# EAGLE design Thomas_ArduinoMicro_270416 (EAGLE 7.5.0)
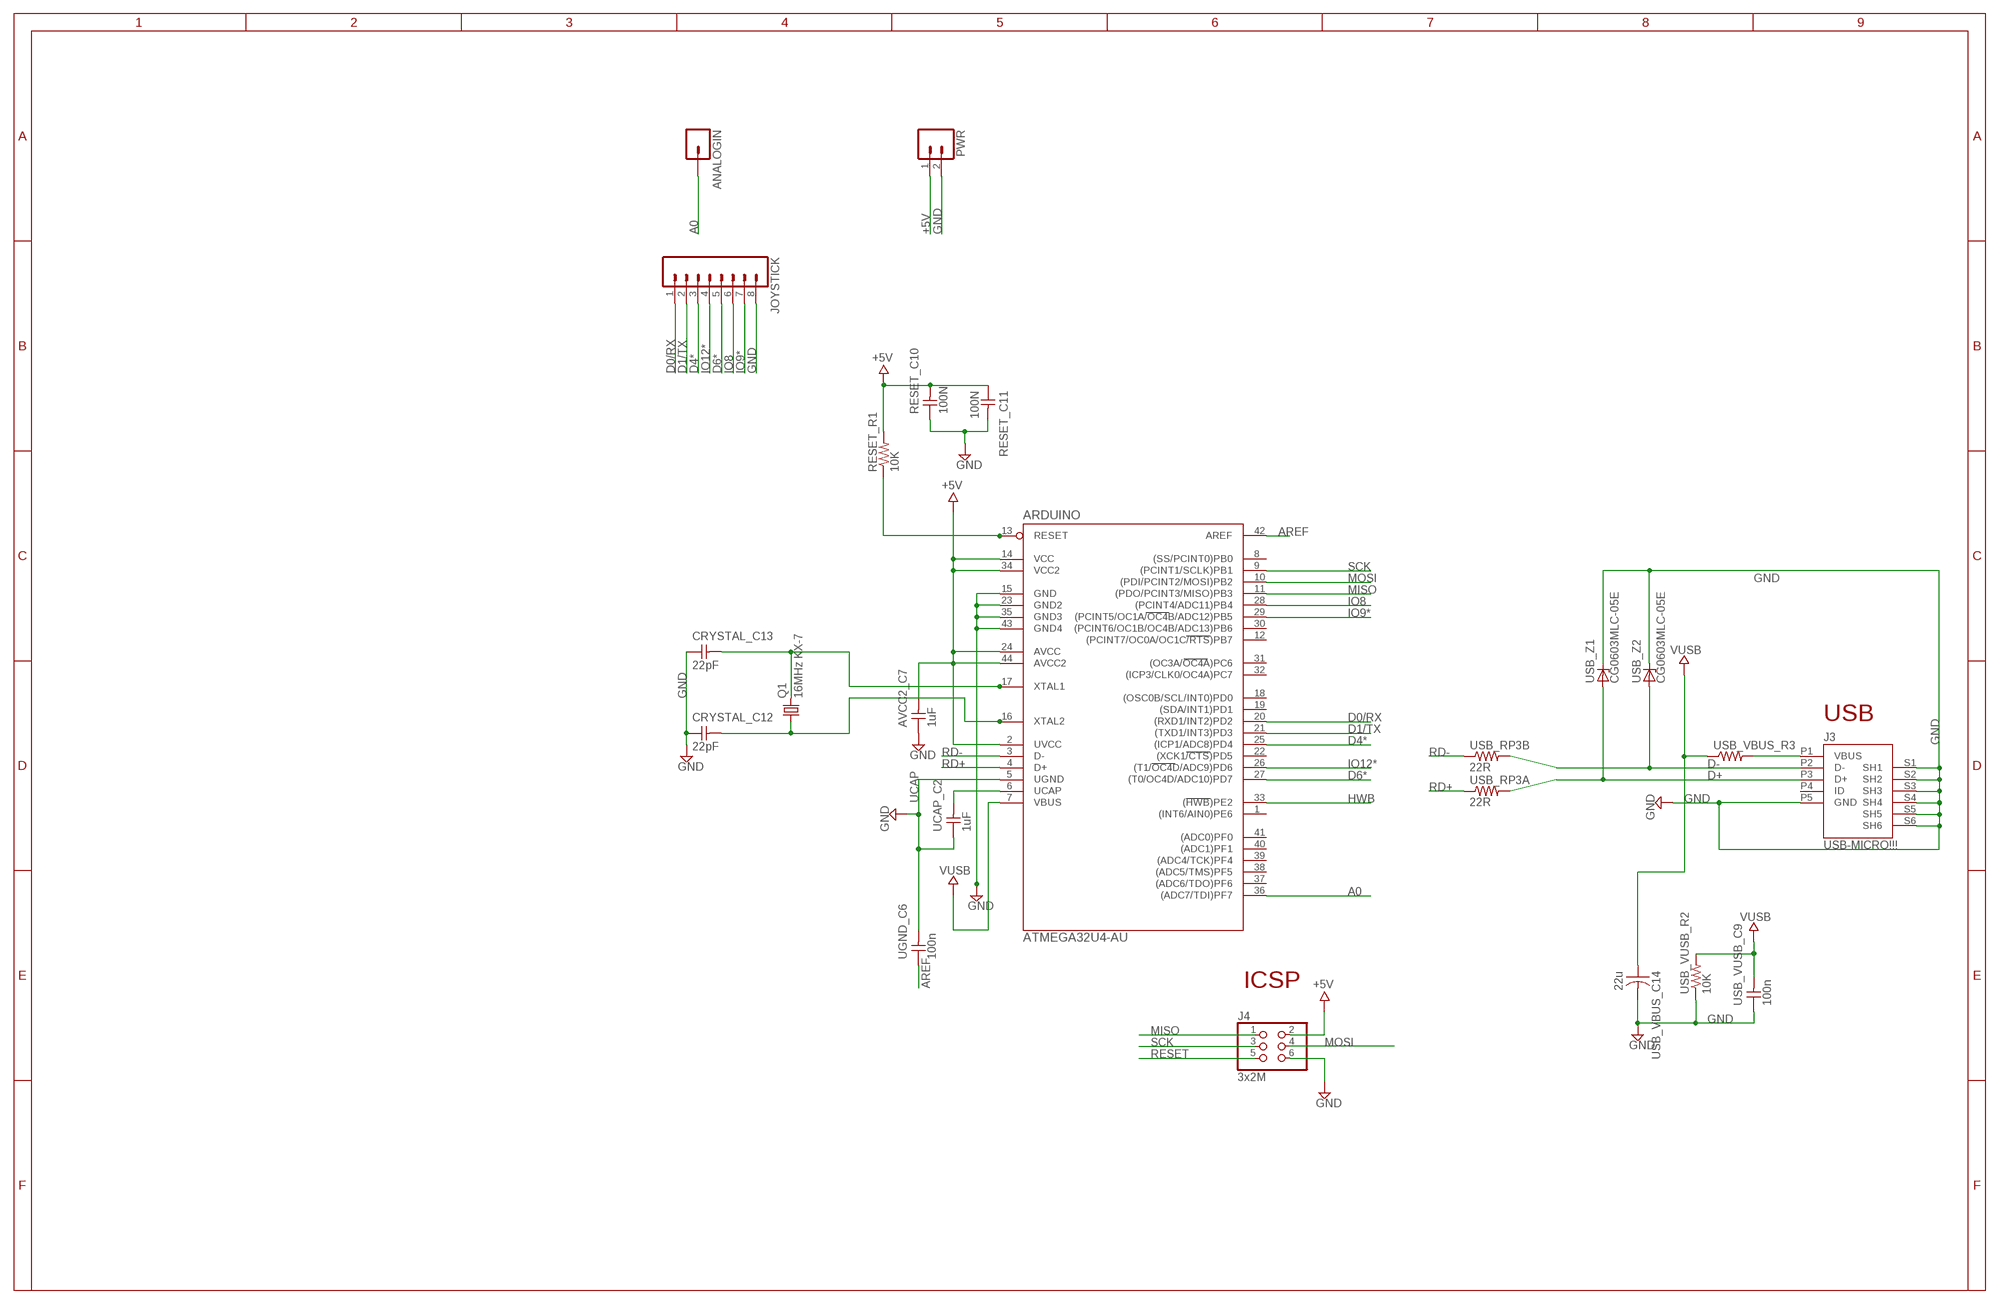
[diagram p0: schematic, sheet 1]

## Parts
ANALOGIN  M01PTH_LONGPAD  [1X01_LONGPAD]
ARDUINO  ATMEGA32U4-AU  [TQFP44]
AVCC2_C7  1uF  CAP-UNPOLARIZEDFAB  [C1206FAB]
CRYSTAL_C12  22pF  CAP-UNPOLARIZEDFAB  [C1206FAB]
CRYSTAL_C13  22pF  CAP-UNPOLARIZEDFAB  [C1206FAB]
J3  USB-MICRO!!!  MYCON2_USB-MINI-B  [CON2_USB_MICRO_B_AT]
J4  3x2M  PINHD-2X3  [2X03]
JOYSTICK  M08LONGPADS  [1X08_LONGPADS]
PWR  M02PTH3  [1X02_LONGPADS]
Q1  16MHz KX-7  CSM-7X-DU  [CSM-7X-DU]
RESET_C10  100N  CAP-UNPOLARIZEDFAB  [C1206FAB]
RESET_C11  100N  CAP-UNPOLARIZEDFAB  [C1206FAB]
RESET_R1  10K  RESISTOR1206  [1206]
UCAP_C2  1uF  CAP-UNPOLARIZEDFAB  [C1206FAB]
UGND_C6  100n  CAP-UNPOLARIZEDFAB  [C1206FAB]
USB_RP3A  22R  RESISTOR1206  [1206]
USB_RP3B  22R  RESISTOR1206  [1206]
USB_VBUS_C14  22u  CAP-US1206FAB  [C1206FAB]
USB_VBUS_R3  RESISTOR1206  [1206]
USB_VUSB_C9  100n  CAP-UNPOLARIZEDFAB  [C1206FAB]
USB_VUSB_R2  10K  RESISTOR1206  [1206]
USB_Z1  CG0603MLC-05E  ZENER_DIODESOD123  [SOD123]
USB_Z2  CG0603MLC-05E  ZENER_DIODESOD123  [SOD123]

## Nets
+5V: ARDUINO.2(UVCC) ARDUINO.14(VCC) ARDUINO.24(AVCC) ARDUINO.34(VCC2) ARDUINO.44(AVCC2) AVCC2_C7.2 J4.2 PWR.1
A0: ANALOGIN.1 ARDUINO.36((ADC7/TDI)PF7)
AREF: ARDUINO.42(AREF) UGND_C6.1
C11: RESET_C10.2 RESET_C11.1 RESET_R1.2 ; supply symbol labelled +5V
D0/RX: ARDUINO.20((RXD1/INT2)PD2) JOYSTICK.1
D1/TX: ARDUINO.21((TXD1/INT3)PD3) JOYSTICK.2
D4*: ARDUINO.25((ICP1/ADC8)PD4) JOYSTICK.3
D6*: ARDUINO.27((T0/OC4D/ADC10)PD7) JOYSTICK.5
D+: J3.P3(D+) USB_RP3A.2 USB_Z1.ANODE
D-: J3.P2(D-) USB_RP3B.2 USB_Z2.ANODE
GND: ARDUINO.15(GND) ARDUINO.23(GND2) ARDUINO.35(GND3) ARDUINO.43(GND4) AVCC2_C7.1 CRYSTAL_C12.1 CRYSTAL_C13.1 J3.P5(GND) J3.S1(SH1) J3.S2(SH2) J3.S3(SH3) J3.S4(SH4) J3.S5(SH5) J3.S6(SH6) J4.6 JOYSTICK.8 PWR.2 RESET_C10.1 RESET_C11.2 USB_VBUS_C14.2 USB_VUSB_C9.1 USB_VUSB_R2.1 USB_Z1.CATHODE USB_Z2.CATHODE
HWB: ARDUINO.33((HWB)PE2)
IO8: ARDUINO.28((PCINT4/ADC11)PB4) JOYSTICK.6
IO9*: ARDUINO.29((PCINT5/OC1A/OC4B/ADC12)PB5) JOYSTICK.7
IO12*: ARDUINO.26((T1/OC4D/ADC9)PD6) JOYSTICK.4
MISO: ARDUINO.11((PDO/PCINT3/MISO)PB3) J4.1
MOSI: ARDUINO.10((PDI/PCINT2/MOSI)PB2) J4.4
N$1: ARDUINO.13(RESET) RESET_R1.1
N$2: ARDUINO.6(UCAP) UCAP_C2.2
N$3: ARDUINO.16(XTAL2) CRYSTAL_C12.2 Q1.1
N$4: ARDUINO.17(XTAL1) CRYSTAL_C13.2 Q1.2
N$5: J3.P1(VBUS) USB_VBUS_R3.2
RD+: ARDUINO.4(D+) USB_RP3A.1
RD-: ARDUINO.3(D-) USB_RP3B.1
RESET: J4.5
SCK: ARDUINO.9((PCINT1/SCLK)PB1) J4.3
UCAP: ARDUINO.5(UGND) UCAP_C2.1 UGND_C6.2 ; supply symbol labelled GND
VUSB: ARDUINO.7(VBUS) USB_VBUS_C14.1 USB_VBUS_R3.1 USB_VUSB_C9.2 USB_VUSB_R2.2
Unconnected: ARDUINO.1((INT6/AIN0)PE6) ARDUINO.8((SS/PCINT0)PB0) ARDUINO.12((PCINT7/OC0A/OC1C/RTS)PB7) ARDUINO.18((OSC0B/SCL/INT0)PD0) ARDUINO.19((SDA/INT1)PD1) ARDUINO.22((XCK1/CTS)PD5) ARDUINO.30((PCINT6/OC1B/OC4B/ADC13)PB6) ARDUINO.31((OC3A/OC4A)PC6) ARDUINO.32((ICP3/CLK0/OC4A)PC7) ARDUINO.37((ADC6/TDO)PF6) ARDUINO.38((ADC5/TMS)PF5) ARDUINO.39((ADC4/TCK)PF4) ARDUINO.40((ADC1)PF1) ARDUINO.41((ADC0)PF0) J3.P4(ID)

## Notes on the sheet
- USB
- ICSP

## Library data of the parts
ANALOGIN = SparkFun-Connectors:M01: Header 1
ARDUINO = mega32U4:ATMEGA32U4-AU
AVCC2_C7 CRYSTAL_C12 CRYSTAL_C13 RESET_C10 RESET_C11 UCAP_C2 UGND_C6 USB_VUSB_C9 = fab:CAP-UNPOLARIZED
J3 = SmartPrj:MYCON2_USB-MINI-B
J4 = SmartPrj:PINHD-2X3: PIN HEADER
JOYSTICK = SparkFun-Connectors:M08: Header 8 Standard 8-pin 0.1" header. Use with straight break away headers (SKU : PRT-00116), right angle break away headers (PRT-00553), swiss pins (PRT-00743), machine pins (PRT-00117), and female headers (PRT-00115).
PWR = SparkFun-Connectors:M02: Standard 2-pin 0.1" header. Use with
Q1 = FAB_Hello:CSM-7X-DU: SMD CRYSTAL; OC_FARNELL: unknown; OC_NEWARK: unknown
RESET_R1 USB_RP3A USB_RP3B USB_VBUS_R3 USB_VUSB_R2 = SparkFun-Passives:RESISTOR: Resistor
USB_VBUS_C14 = fab:CAP-US
USB_Z1 USB_Z2 = fab:ZENER_DIODE: zener diode

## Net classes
0 default: width 0.254 mm, drill 0.61 mm, clearance 0.203 mm

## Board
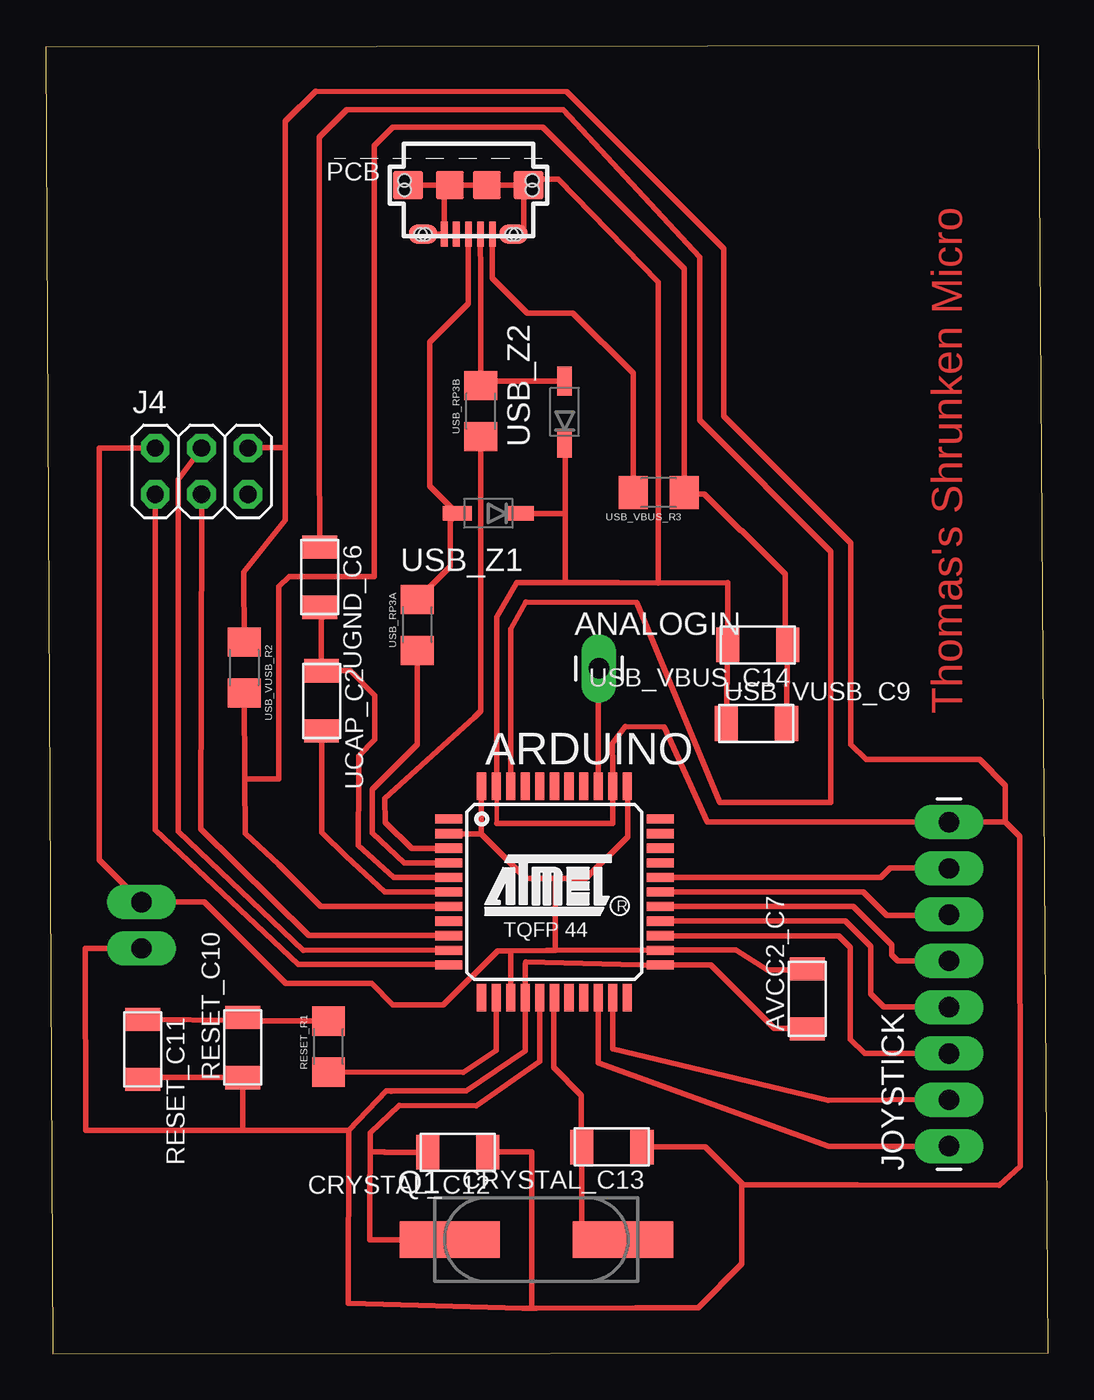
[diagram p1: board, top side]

Size 54.99 x 71.8 mm. Coordinates in mm from the lower left corner, seen from the top.
Outline: 0.38,0 54.99,0.08 54.48,71.8 0,71.69 0.38,0
Copper layers (1*16): Top 0.035mm / dielectric 1.5mm / Bottom 0.035mm
Design rules "default": minimum track width 10mil, minimum drill 24mil, track to track 8mil, track to pad 8mil, pad to pad 8mil, via to via 8mil, smd to smd 8mil, copper to edge 40mil, drill to drill 8mil, minimum pad ring 10mil, minimum via ring 8mil, stop-mask expansion 4mil, vias tented up to drill 0mil, thermal gap 10mil

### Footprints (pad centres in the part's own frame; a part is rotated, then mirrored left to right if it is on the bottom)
1X01_LONGPAD = drill 1.118 pad 1.88 long: 1 0,0
TQFP44 = smd 1.5 x 0.5: 1 -5.8,4; 2 -5.8,3.2; 3 -5.8,2.4; 4 -5.8,1.6; 5 -5.8,0.8; 6 -5.8,0; 7 -5.8,-0.8; 8 -5.8,-1.6; 9 -5.8,-2.4; 10 -5.8,-3.2; 11 -5.8,-4; 23 5.8,-4; 24 5.8,-3.2; 25 5.8,-2.4; 26 5.8,-1.6; 27 5.8,-0.8; 28 5.8,0; 29 5.8,0.8; 30 5.8,1.6; 31 5.8,2.4; 32 5.8,3.2; 33 5.8,4 | smd 0.5 x 1.5: 12 -4,-5.8; 13 -3.2,-5.8; 14 -2.4,-5.8; 15 -1.6,-5.8; 16 -0.8,-5.8; 17 0,-5.8; 18 0.8,-5.8; 19 1.6,-5.8; 20 2.4,-5.8; 21 3.2,-5.8; 22 4,-5.8; 34 4,5.8; 35 3.2,5.8; 36 2.4,5.8; 37 1.6,5.8; 38 0.8,5.8; 39 0,5.8; 40 -0.8,5.8; 41 -1.6,5.8; 42 -2.4,5.8; 43 -3.2,5.8; 44 -4,5.8
C1206FAB = smd 1.27 x 1.905: 1 -1.651,0; 2 1.651,0
CON2_USB_MICRO_B_AT = smd 0.406 x 1.346: P1 -1.321,2.692; P2 -0.66,2.692; P3 0,2.692; P4 0.66,2.692; P5 1.321,2.692 | smd 1.651 x 1.549: S1 -3.302,0; S2 3.302,0 | smd 1.524 x 1.016: S3 -2.489,2.692; S4 2.489,2.692 | smd 1.524 x 1.524: S5 -1.016,0; S6 1.016,0 | hole 0.7: -3.505,0.254; -3.505,-0.254; 3.505,0.254; 3.505,-0.254; -2.616,2.692; -2.362,2.692; 2.362,2.692; 2.616,2.692
2X03 = drill 0.95 pad 1.55 octagon: 1 -2.54,-1.27; 2 -2.54,1.27; 3 0,-1.27; 4 0,1.27; 5 2.54,-1.27; 6 2.54,1.27
1X08_LONGPADS = drill 1.118 pad 1.88 long: 1 0,0; 2 2.54,0; 3 5.08,0; 4 7.62,0; 5 10.16,0; 6 12.7,0; 7 15.24,0; 8 17.78,0
1X02_LONGPADS = drill 1.118 pad 1.88 long: 1 0,0; 2 2.54,0
CSM-7X-DU = smd 5.5 x 2: 1 -4.75,0; 2 4.75,0
1206 = smd 1.6 x 1.8: 1 -1.4,0; 2 1.4,0
SOD123 = smd 1.6 x 0.8: ANODE 1.7,0; CATHODE -1.7,0

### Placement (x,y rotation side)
ANALOGIN  30.35,37.62 0 top
ARDUINO  27.91,25.35 0 top
AVCC2_C7  41.78,19.48 90 top
CRYSTAL_C12  22.61,11.07 180 top
CRYSTAL_C13  31.06,11.35 180 top
J3  23.19,64.14 180 top
J4  8.56,48.44 0 top
JOYSTICK  49.56,11.4 90 top
PWR  5.26,24.79 270 top
Q1  26.92,6.27 0 top
RESET_C10  10.82,16.81 90 top
RESET_C11  5.33,16.71 270 top
RESET_R1  15.52,16.87 90 top
UCAP_C2  15.14,35.84 270 top
UGND_C6  15.04,42.62 270 top
USB_RP3A  20.4,40.01 90 top
USB_RP3B  23.88,51.74 90 top
USB_VBUS_C14  39.07,38.91 180 top
USB_VBUS_R3  33.63,47.27 180 top
USB_VUSB_C9  38.99,34.59 0 top
USB_VUSB_R2  10.9,37.67 270 top
USB_Z1  24.28,46.13 180 top
USB_Z2  28.47,51.69 90 top

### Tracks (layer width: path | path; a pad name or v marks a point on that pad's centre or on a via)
+5V
  Top 0.254: 22.83,28.52 22.2,28.52 ARDUINO.2 | 23.91,31.04 ARDUINO.44 | 25.51,19.69 ARDUINO.14 | 33.63,22.17 ARDUINO.24
  Top 0.305: 25.51,22.12 25.51,19.69 | 33.63,22.17 27.5,22.15 | 27.5,22.15 25.51,22.12 | AVCC2_C7.2 41.73,21.08 39.57,21.08 37.87,22.17 33.74,22.17 ARDUINO.24 | J4.2 2.95,49.71 2.95,27.1 PWR.1 8.71,24.79 13.18,20.32 17.88,20.32 19.05,19.15 21.82,19.15 24.79,22.12 25.51,22.12 | 23.91,31.04 23.9,31.03 23.9,28.52 | 22.83,28.52 23.9,28.52 | 27.5,22.15 27.97,22.15 27.97,26.06 | ARDUINO.34 31.93,31.15 31.93,28.37 29.64,26.09 27.99,26.09 27.97,26.06 | 23.9,28.52 26.34,26.09 27.94,26.09 27.97,26.06
A0
  Top 0.305: ARDUINO.36 30.31,37.58 ANALOGIN.1
AREF
  Top 0.305: ARDUINO.42 25.51,39.79 26.34,41.25 32.44,41.22 36.98,30.25 43.08,30.25 43.08,44.04 35.89,51.23 35.89,60.2 28.4,68.28 16.51,68.28 15.01,66.78 15.01,49.86 | UGND_C6.1 15.01,49.86 | 15.01,49.86 15.01,50.11
C11
  Top 0.305: RESET_R1.2 11.02,18.27 RESET_C10.2 10.67,18.31 RESET_C11.1
D0/RX
  Top 0.305: ARDUINO.20 30.31,15.96 42.95,11.38 JOYSTICK.1
D1/TX
  Top 0.305: ARDUINO.21 31.11,16.74 42.93,13.92 49.53,13.97 JOYSTICK.2
D4*
  Top 0.305: ARDUINO.25 43.5,22.95 44.15,22.3 44.15,17.27 44.93,16.48 JOYSTICK.3
D6*
  Top 0.305: ARDUINO.27 44.31,24.55 46.41,22.45 46.41,21.9 46.74,21.56 JOYSTICK.5
D+
  Top 0.305: J3.P3 23.19,57.63 21.08,55.52 21.08,47.63 USB_Z1.ANODE 22.2,45.74 22.2,43.21 USB_RP3A.2
D-
  Top 0.305: J3.P2 23.86,58.98 23.86,58.77 USB_RP3B.2 23.88,53.39 USB_Z2.ANODE
GND
  Top 0.254: 26.33,19.63 ARDUINO.15 | 33.63,21.32 ARDUINO.23 | 24.74,29.11 24.74,31.06 ARDUINO.43 24.74,31.38 | 31.09,30.43 31.09,31.06 ARDUINO.35 31.09,31.38
  Top 0.305: 24.74,29.11 31.11,29.11 31.11,30.43 31.09,30.43 | 24.74,31.38 24.74,40.44 25.86,42.32 28.47,42.32 | 31.09,31.38 31.1,32.26 31.09,33.5 31.8,34.42 33.93,34.42 36.3,29.18 JOYSTICK.8 52.65,29.18 | J3.S4 J3.P5 21.87,63.83 J3.S6 | J3.S2 J3.S6 | 10.82,12.27 RESET_C10.1 5.44,15.16 RESET_C11.2 | 10.82,12.27 2.21,12.28 2.18,22.26 PWR.2 | 26.92,2.52 32.38,2.54 35.79,2.54 38.19,4.94 38.19,9.4 | 26.92,2.52 26.16,2.51 16.61,2.77 16.62,12.28 | J3.S6 J3.S5 J3.S1 | ARDUINO.23 33.73,21.36 36.5,21.36 36.5,21.34 39.98,17.86 41.76,17.86 AVCC2_C7.1 | 23.09,14.43 26.31,16.64 ARDUINO.15 | 23.09,14.43 18.95,14.4 | 44.02,9.27 44.53,9.27 | 44.53,9.27 52.32,9.25 53.47,10.29 53.44,28.14 53.44,28.39 52.65,29.18 | 28.47,42.32 31.42,42.32 33.6,42.3 | 23.09,14.43 18.69,14.43 16.62,12.28 | USB_VUSB_C9.1 USB_VBUS_C14.2 37.41,42.32 33.6,42.3 | 10.82,12.27 10.78,12.28 16.62,12.28 | 13.16,49.73 13.16,67.64 14.81,69.29 28.6,69.27 37.21,60.66 37.21,51.46 44.17,44.5 44.17,33.45 45.01,32.61 51.23,32.61 52.65,31.2 52.65,29.18 | 13.16,49.73 13.16,45.77 10.87,42.9 USB_VUSB_R2.1 | 44.53,9.27 44.52,9.27 38.32,9.27 38.19,9.4 | 33.6,42.3 33.6,58.8 33.61,58.8 28.12,64.47 26.96,64.47 26.63,64.14 J3.S1 | 38.19,9.4 38.13,9.4 38.13,9.42 36.19,11.35 CRYSTAL_C13.1 | J3.S1 26.24,63.88 26.24,61.44 J3.S3 | J4.6 11.13,49.73 13.16,49.73 | CRYSTAL_C12.1 24.26,11.1 26.67,11.1 26.67,2.52 26.92,2.52 | ARDUINO.15 26.31,21.41 26.33,21.5 33.63,21.32 | ARDUINO.15 | USB_Z2.CATHODE 28.5,49.99 28.5,46.13 | 28.5,46.13 28.5,42.34 28.47,42.32 | USB_Z1.CATHODE 28.5,46.13
  Top 0.406: USB_Z2.CATHODE
IO8
  Top 0.305: ARDUINO.28 44.86,25.35 46.15,24.05 49.5,24.05 JOYSTICK.6
IO9*
  Top 0.305: ARDUINO.29 45.81,26.15 46.33,26.67 49.53,26.67 JOYSTICK.7
IO12*
  Top 0.254: 33.95,23.76 ARDUINO.26
  Top 0.305: 33.95,23.76 43.85,23.76 45.26,22.35 45.26,19.76 45.97,19.05 49.53,19.05 JOYSTICK.4
MISO
  Top 0.254: 21.96,21.39 ARDUINO.11
  Top 0.305: 21.96,21.39 13.86,21.39 6.02,28.77 J4.1
MOSI
  Top 0.254: 21.88,22.17 ARDUINO.10
  Top 0.305: 21.88,22.17 14.12,22.15 7.29,28.68 7.29,47.98 J4.4
N$1
  Top 0.305: RESET_R1.1 22.91,15.44 24.71,16.66 ARDUINO.13 | ARDUINO.13
N$2
  Top 0.305: ARDUINO.6 18.59,25.35 16.48,27.32 15.14,28.63 UCAP_C2.2
N$3
  Top 0.305: ARDUINO.16 27.11,16.07 23.62,13.61 19.41,13.64 17.81,12.14 17.8,11.08 | Q1.1 17.78,6.27 17.78,7.34 17.78,8.64 17.8,11.08 | CRYSTAL_C12.2 18.59,11.07 18.59,11.08 17.8,11.08
N$4
  Top 0.305: ARDUINO.17 27.86,19.5 27.86,15.72 29.39,14.2 29.39,11.38 CRYSTAL_C13.2 29.41,6.66 29.79,6.27 Q1.2
N$5
  Top 0.305: J3.P1 24.51,59.03 26.42,57.12 28.93,57.12 32.23,53.83 USB_VBUS_R3.2
RD+
  Top 0.305: ARDUINO.4 20.83,26.95 19.68,26.95 17.91,28.6 17.93,30.99 20.4,33.45 USB_RP3A.1
RD-
  Top 0.305: ARDUINO.3 20.08,27.75 18.64,29.16 18.62,30.48 23.52,34.93 23.88,35.28 USB_RP3B.1
SCK
  Top 0.254: 21.88,22.97 ARDUINO.9
  Top 0.305: 21.88,22.97 14.43,22.97 8.51,28.82 8.56,46.2 J4.3
UCAP
  Top 0.305: ARDUINO.5 19.09,26.15 17.14,27.91 17.17,31.62 17.17,32.82 18.06,33.71 18.06,36.14 16.71,37.49 UCAP_C2.1 15.14,37.56 15.13,37.57 | UGND_C6.2 15.85,40.51 15.75,40.61 15.75,40.84 15.11,40.34 15.11,38.28 15.13,37.57 | 15.13,37.57 15.14,37.29 15.11,37.26
VUSB
  Top 0.305: ARDUINO.7 15.1,24.55 12.79,26.86 10.95,28.55 10.93,31.54 | USB_VUSB_R2.2 10.93,31.54 | USB_VUSB_C9.2 USB_VBUS_C14.1 40.56,39.07 40.56,42.8 38.18,45.19 38.13,45.19 36.12,47.19 35.11,47.19 USB_VBUS_R3.1 35.03,59.56 27.28,67.31 19.05,67.31 18.03,66.29 18.03,42.65 17.35,42.65 13.36,42.67 12.79,42.1 12.79,31.54 10.93,31.54

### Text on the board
Top: Thomas's Shrunken Micro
